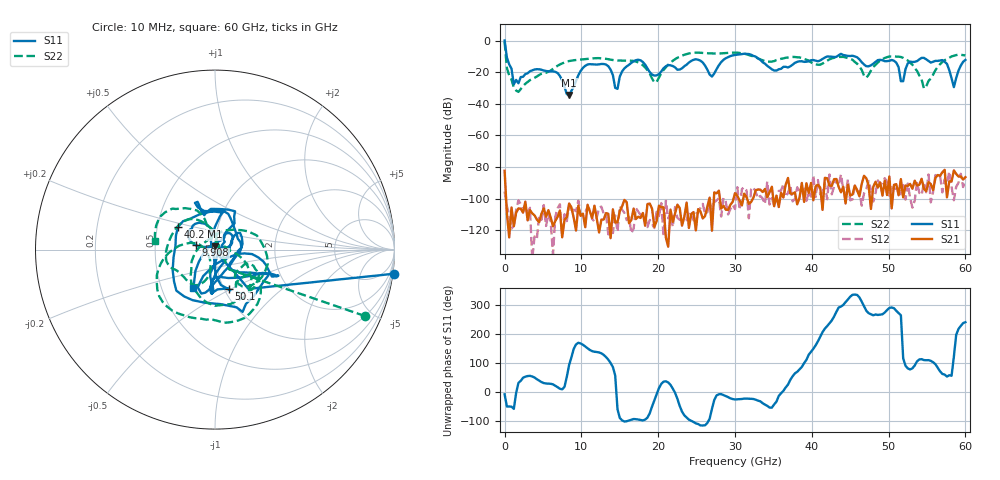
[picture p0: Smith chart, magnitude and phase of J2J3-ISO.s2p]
!Keysight Technologies,N5227A,US51270214,A.10.65.11
!Date: Thursday, October 15, 2020 08:22:51
!Correction: S11(Full 2 Port(1,2))
!S21(Full 2 Port(1,2))
!S12(Full 2 Port(1,2))
!S22(Full 2 Port(1,2))
!S2P File: Measurements: S11, S21, S12, S22:
# Hz S  dB  R 50
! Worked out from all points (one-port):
!   201 points, 10 MHz to 60 GHz, reference 50 ohm
!   lowest |S11| = -34.5 dB at 8.409 GHz (marker M1), VSWR 1.04, Z = 49.9 + j1.88 ohm
!   |S11| at or under -10 dB: 287.2 MHz to 29.33 GHz (29.04 GHz wide, 196 % of centre); 32.58 GHz to 43.29 GHz (10.71 GHz wide, 28.2 % of centre); 45.57 GHz to end of sweep
!   S11 on the Smith chart (normalised r, x): 10 MHz: -1, -15; 9.908 GHz: 0.81, +0.04; 40.2 GHz: 0.64, +0.17; 50.1 GHz: 1.05, -0.48; 60 GHz: 0.72, -0.33
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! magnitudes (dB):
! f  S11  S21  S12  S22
! 10 MHz  0.1  -82.3  -95.5  -0.8
! 309.9 MHz  -10.8  -109.2  -104.8  -17.4
! 1.81 GHz  -27.0  -106.1  -100.9  -32.5
! 6.609 GHz  -19.8  -114.0  -111.3  -16.9
! 8.409 GHz  -34.5  -103.0  -104.2  -13.0
! 9.908 GHz  -19.2  -110.8  -110.6  -12.0
! 10.21 GHz  -17.2  -109.4  -110.4  -11.9
! 13.21 GHz  -15.2  -109.0  -109.4  -11.5
! 14.71 GHz  -30.5  -114.8  -120.7  -12.6
! 17.11 GHz  -12.4  -112.8  -105.9  -13.3
! 20.11 GHz  -21.3  -104.4  -110.9  -23.5
! 24.91 GHz  -11.8  -120.0  -109.3  -7.6
! 27.01 GHz  -22.8  -120.2  -107.0  -8.1
! 30 GHz  -9.1  -96.4  -106.5  -7.6
! 40.2 GHz  -12.3  -101.0  -85.4  -14.8
! 47.1 GHz  -16.3  -87.1  -93.9  -23.5
! 50.1 GHz  -12.8  -85.9  -98.2  -10.1
! 51.9 GHz  -25.7  -99.1  -91.3  -11.0
! 54.6 GHz  -11.0  -93.7  -89.8  -30.3
! 57.6 GHz  -14.8  -99.1  -90.4  -11.6
! 58.5 GHz  -29.5  -82.1  -100.9  -9.6
! 60 GHz  -12.3  -86.3  -87.9  -9.4
